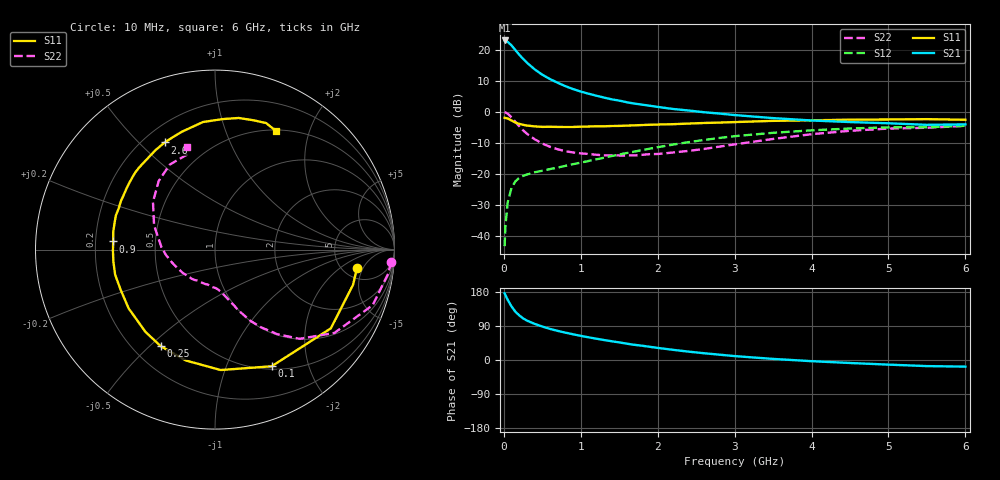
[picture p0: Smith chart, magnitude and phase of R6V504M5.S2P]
! SIEMENS Small Signal Semiconductors
! BFR193
! Si NPN RF Bipolar Junction Transistor in SOT23
! VCE = 0.5 V  IC = 4.5 mA
! Common Emitter S-Parameters:  May  1996
# GHz  S  MA  R  50
!  f  S11  S21  S12  S22
! GHz  MAG  ANG  MAG  ANG  MAG  ANG  MAG  ANG
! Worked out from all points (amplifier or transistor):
!   36 points, 10 MHz to 6 GHz, reference 50 ohm
!   highest |S21| = 22.9 dB at 10 MHz (marker M1)
!   |S21| within 3 dB of that: start of sweep to 146.7 MHz
!   unconditionally stable (mu >= 1): 867.2 MHz to 2.461 GHz; 5.351 GHz to end of sweep
!   at 250 MHz: K = 0.41, MSG = 18.8 dB, |S12| = -20.6 dB
!   at 1.4 GHz: K = 1.10, MAG = 7.2 dB, |S12| = -14.3 dB
!   at 6 GHz: K = 1.00, MAG = -0.2 dB, |S12| = -4.5 dB
!   S11 on the Smith chart (normalised r, x): 10 MHz: 6.80, -3.75; 100 MHz: 0.54, -1.46; 250 MHz: 0.31, -0.54; 900 MHz: 0.28, +0.04; 2.6 GHz: 0.28, +0.60; 6 GHz: 0.51, +1.51
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0.01  0.798 -7.2  14.01 175.9  0.0069 86.4  0.9855 -4.0
0.02  0.7937 -14.3  13.99 171.2  0.0143 81.5  0.9736 -8.0
0.05  0.7805 -34.2  13.3 158.9  0.0348 72.8  0.9316 -19.4
0.1  0.7226 -64.1  11.67 141.3  0.06 59.6  0.8113 -34.9
0.15  0.6718 -87.3  9.8 127.5  0.0759 50.4  0.6852 -46.5
0.2  0.6388 -104.7  8.292 117.8  0.0866 45.2  0.5861 -53.6
0.25  0.6171 -119.4  7.091 109.9  0.0933 41.8  0.5038 -59.3
0.3  0.6002 -130.2  6.146 104.1  0.0978 39.9  0.443 -63.6
0.4  0.5821 -145.8  4.813 95.4  0.1063 38.4  0.3617 -69.0
0.5  0.5714 -156.9  3.935 88.3  0.1127 38.6  0.3088 -72.8
0.6  0.5737 -165.9  3.357 82.1  0.1197 39.8  0.273 -76.7
0.7  0.5701 -173.4  2.923 76.8  0.1267 41.4  0.2494 -80.0
0.9  0.569 175.4  2.317 67.8  0.1437 43.8  0.2216 -86.0
1.1  0.579 165.1  1.952 59.9  0.1615 46.1  0.2095 -93.4
1.3  0.5835 156.7  1.694 52.8  0.1824 47.6  0.199 -101.8
1.6  0.5987 145.6  1.42 43.0  0.2174 48.4  0.1981 -115.5
2.2  0.631 126.8  1.108 26.8  0.2966 45.2  0.2213 -143.8
2.6  0.6596 115.2  0.983 17.9  0.3516 40.7  0.2519 -164.1
3.5  0.7139 95.4  0.79 2.9  0.4588 26.9  0.3653 158.3
4.5  0.7452 79.8  0.683 -7.9  0.5378 11.4  0.4943 129.4
5.5  0.7604 68.0  0.616 -16.1  0.5632 -3.1  0.5527 106.0
6  0.7435 62.9  0.627 -17.5  0.5948 -7.4  0.5929 105.1
